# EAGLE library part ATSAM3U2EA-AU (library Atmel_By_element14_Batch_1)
AT91ARM Cortex M3-based Microcontrollers
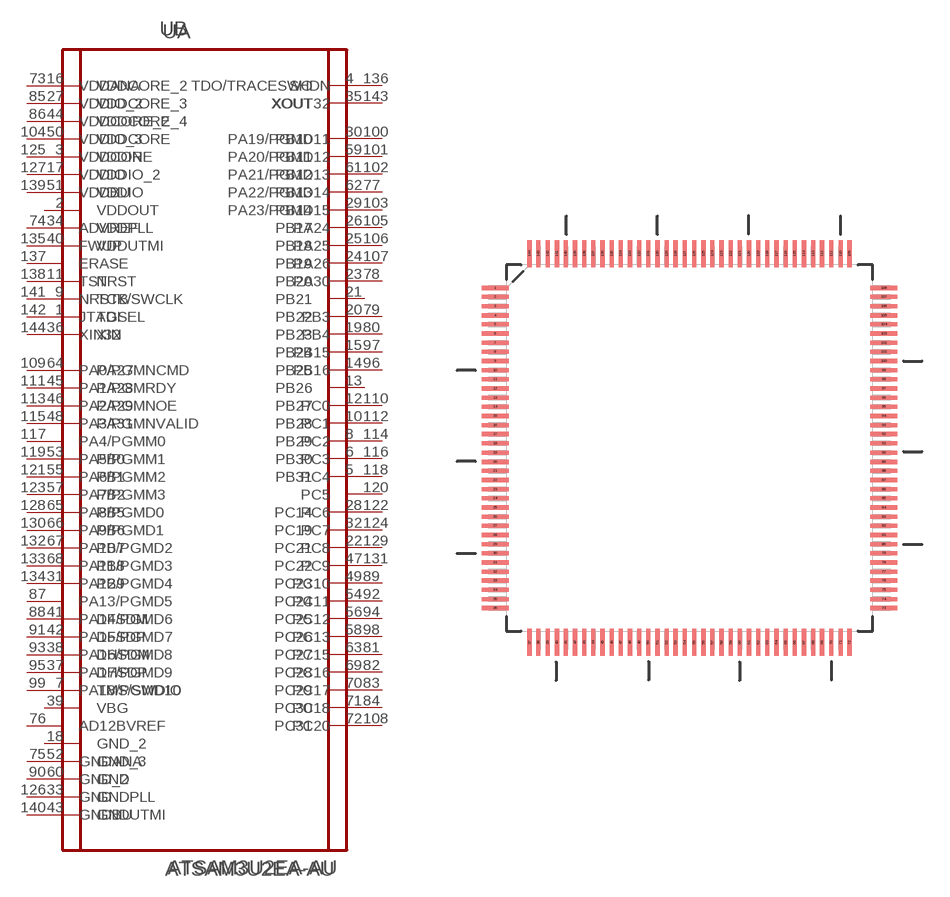
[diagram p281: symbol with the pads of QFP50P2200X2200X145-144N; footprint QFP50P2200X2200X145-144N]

Designator prefix U; gates A=ATSAM3U2EA-AU_A B=ATSAM3U2EA-AU_B

## ATSAM3U2EA-AU (DESCRIPTION: AT91ARM Cortex M3-based Microcontrollers; MPN: ATSAM3U2EA-AU; OC_FARNELL: 1841663; OC_NEWARK: 12T1319; PACKAGE: LQFP-144; SUPPLIER: Atmel Corporation)  [QFP50P2200X2200X145-144N]
1  A:TDI  in
2  A:VDDOUT  pwr
3  A:VDDIN  pwr
4  A:TDO/TRACESWO  out
5  A:PB31
6  A:PB30
7  A:TMS/SWDIO
8  A:PB29
9  A:TCK/SWCLK  in
10  A:PB28
11  A:NRST  in
12  A:PB27
13  A:PB26
14  A:PB25
15  A:PB24
16  A:VDDCORE_2  pwr
17  A:VDDIO_2  pwr
18  A:GND_2  pas
19  A:PB23
20  A:PB22
21  A:PB21
22  A:PC21
23  A:PB20
24  A:PB19
25  A:PB18
26  A:PB17
27  A:VDDCORE_3  pwr
28  A:PC14
29  A:PB14
30  A:PB10
31  A:PB9
32  A:PC19
33  A:GNDPLL  pas
34  A:VDDPLL  pwr
35  A:XOUT  out
36  A:XIN  in
37  A:DHSDP
38  A:DHSDM
39  A:VBG
40  A:VDDUTMI  pwr
41  A:DFSDM
42  A:DFSDP
43  A:GNDUTMI  pas
44  A:VDDCORE_4  pwr
45  A:PA28
46  A:PA29
47  A:PC22
48  A:PA31
49  A:PC23
50  A:VDDCORE  pwr
51  A:VDDIO  pwr
52  A:GND_3  pas
53  A:PB0
54  A:PC24
55  A:PB1
56  A:PC25
57  A:PB2
58  A:PC26
59  A:PB11
60  A:GND  pas
61  A:PB12
62  A:PB13
63  A:PC27
64  A:PA27
65  A:PB5
66  A:PB6
67  A:PB7
68  A:PB8
69  A:PC28
70  A:PC29
71  A:PC30
72  A:PC31
73  B:VDDANA  pwr
74  B:ADVREF  in
75  B:GNDANA  pas
76  B:AD12BVREF  pas
77  B:PA22/PGMD14
78  B:PA30
79  B:PB3
80  B:PB4
81  B:PC15
82  B:PC16
83  B:PC17
84  B:PC18
85  B:VDDIO_2  pwr
86  B:VDDCORE_2  pwr
87  B:PA13/PGMD5
88  B:PA14/PGMD6
89  B:PC10
90  B:GND_2  pas
91  B:PA15/PGMD7
92  B:PC11
93  B:PA16/PGMD8
94  B:PC12
95  B:PA17/PGMD9
96  B:PB16
97  B:PB15
98  B:PC13
99  B:PA18/PGMD10
100  B:PA19/PGMD11
101  B:PA20/PGMD12
102  B:PA21/PGMD13
103  B:PA23/PGMD15
104  B:VDDIO_3  pwr
105  B:PA24
106  B:PA25
107  B:PA26
108  B:PC20
109  B:PA0/PGMNCMD
110  B:PC0
111  B:PA1/PGMRDY
112  B:PC1
113  B:PA2/PGMNOE
114  B:PC2
115  B:PA3/PGMNVALID
116  B:PC3
117  B:PA4/PGMM0
118  B:PC4
119  B:PA5/PGMM1
120  B:PC5
121  B:PA6/PGMM2
122  B:PC6
123  B:PA7/PGMM3
124  B:PC7
125  B:VDDCORE  pwr
126  B:GND  pas
127  B:VDDIO  pwr
128  B:PA8/PGMD0
129  B:PC8
130  B:PA9/PGMD1
131  B:PC9
132  B:PA10/PGMD2
133  B:PA11/PGMD3
134  B:PA12/PGMD4
135  B:FWUP  in
136  B:SHDN  out
137  B:ERASE  in
138  B:TST  in
139  B:VDDBU  pwr
140  B:GNDBU  pas
141  B:NRSTB  in
142  B:JTAGSEL  in
143  B:XOUT32  out
144  B:XIN32  in

## Footprint QFP50P2200X2200X145-144N (pad centres in mm)
smd 1.473 x 0.229: 1 -10.617,8.738; 2 -10.617,8.255; 3 -10.617,7.747; 4 -10.617,7.239; 5 -10.617,6.756; 6 -10.617,6.248; 7 -10.617,5.74; 8 -10.617,5.258; 9 -10.617,4.75; 10 -10.617,4.242; 11 -10.617,3.759; 12 -10.617,3.251; 13 -10.617,2.743; 14 -10.617,2.261; 15 -10.617,1.753; 16 -10.617,1.245; 17 -10.617,0.762; 18 -10.617,0.254; 19 -10.617,-0.254; 20 -10.617,-0.762; 21 -10.617,-1.245; 22 -10.617,-1.753; 23 -10.617,-2.261; 24 -10.617,-2.743; 25 -10.617,-3.251; 26 -10.617,-3.759; 27 -10.617,-4.242; 28 -10.617,-4.75; 29 -10.617,-5.258; 30 -10.617,-5.74; 31 -10.617,-6.248; 32 -10.617,-6.756; 33 -10.617,-7.239; 34 -10.617,-7.747; 35 -10.617,-8.255; 36 -10.617,-8.738; 73 10.617,-8.738; 74 10.617,-8.255; 75 10.617,-7.747; 76 10.617,-7.239; 77 10.617,-6.756; 78 10.617,-6.248; 79 10.617,-5.74; 80 10.617,-5.258; 81 10.617,-4.75; 82 10.617,-4.242; 83 10.617,-3.759; 84 10.617,-3.251; 85 10.617,-2.743; 86 10.617,-2.261; 87 10.617,-1.753; 88 10.617,-1.245; 89 10.617,-0.762; 90 10.617,-0.254; 91 10.617,0.254; 92 10.617,0.762; 93 10.617,1.245; 94 10.617,1.753; 95 10.617,2.261; 96 10.617,2.743; 97 10.617,3.251; 98 10.617,3.759; 99 10.617,4.242; 100 10.617,4.75; 101 10.617,5.258; 102 10.617,5.74; 103 10.617,6.248; 104 10.617,6.756; 105 10.617,7.239; 106 10.617,7.747; 107 10.617,8.255; 108 10.617,8.738
smd 0.229 x 1.473: 37 -8.738,-10.617; 38 -8.255,-10.617; 39 -7.747,-10.617; 40 -7.239,-10.617; 41 -6.756,-10.617; 42 -6.248,-10.617; 43 -5.74,-10.617; 44 -5.258,-10.617; 45 -4.75,-10.617; 46 -4.242,-10.617; 47 -3.759,-10.617; 48 -3.251,-10.617; 49 -2.743,-10.617; 50 -2.261,-10.617; 51 -1.753,-10.617; 52 -1.245,-10.617; 53 -0.762,-10.617; 54 -0.254,-10.617; 55 0.254,-10.617; 56 0.762,-10.617; 57 1.245,-10.617; 58 1.753,-10.617; 59 2.261,-10.617; 60 2.743,-10.617; 61 3.251,-10.617; 62 3.759,-10.617; 63 4.242,-10.617; 64 4.75,-10.617; 65 5.258,-10.617; 66 5.74,-10.617; 67 6.248,-10.617; 68 6.756,-10.617; 69 7.239,-10.617; 70 7.747,-10.617; 71 8.255,-10.617; 72 8.738,-10.617; 109 8.738,10.617; 110 8.255,10.617; 111 7.747,10.617; 112 7.239,10.617; 113 6.756,10.617; 114 6.248,10.617; 115 5.74,10.617; 116 5.258,10.617; 117 4.75,10.617; 118 4.242,10.617; 119 3.759,10.617; 120 3.251,10.617; 121 2.743,10.617; 122 2.261,10.617; 123 1.753,10.617; 124 1.245,10.617; 125 0.762,10.617; 126 0.254,10.617; 127 -0.254,10.617; 128 -0.762,10.617; 129 -1.245,10.617; 130 -1.753,10.617; 131 -2.261,10.617; 132 -2.743,10.617; 133 -3.251,10.617; 134 -3.759,10.617; 135 -4.242,10.617; 136 -4.75,10.617; 137 -5.258,10.617; 138 -5.74,10.617; 139 -6.248,10.617; 140 -6.756,10.617; 141 -7.239,10.617; 142 -7.747,10.617; 143 -8.255,10.617; 144 -8.738,10.617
